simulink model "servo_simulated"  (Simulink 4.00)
settings: Solver=ode45  StartTime=0.0  StopTime=10  RelTol=1e-3
PreLoadFcn:
  | init_servo
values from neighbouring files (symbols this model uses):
  km = 2.96    [servo_model.m]    (also in init_servo.m; define_simulation_process.m)
libraries: cstblocks x3, simulink3 x3

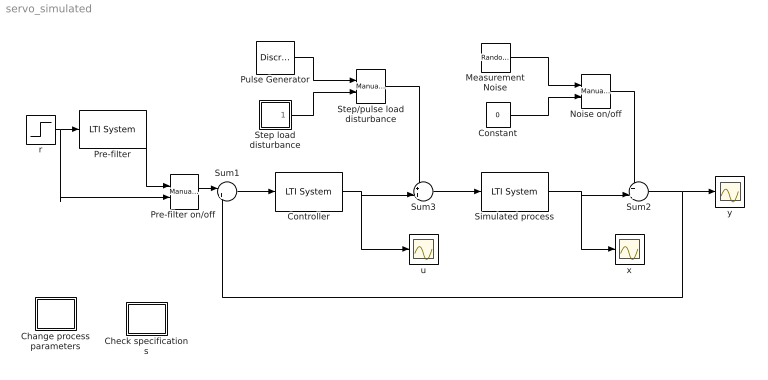
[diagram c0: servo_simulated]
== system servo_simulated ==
  Change process parameters : Subsystem
  Check specifications : Subsystem
  Constant : Constant  Value=0
  Controller : cstblocks/LTI System  sys=C  IC=[]
  Measurement Noise : RandomNumber  Mean=0  Variance=0.05*0.05  Seed=154542  SampleTime=0
  Noise on/off : simulink3/Nonlinear/Manual Switch  sw=1  action=0
  Pre-filter : cstblocks/LTI System  sys=F  IC=[]
  "Pre-filter on/off " : simulink3/Nonlinear/Manual Switch  sw=0  action=0
  Pulse Generator : DiscretePulseGenerator  PulseType=Time-based  Amplitude=-1  Period=100  PulseWidth=0.04  PhaseDelay=5  SampleTime=1
  Simulated process : cstblocks/LTI System  sys=P_sim  IC=[]
  Step load disturbance : Subsystem
  Step/pulse load disturbance : simulink3/Nonlinear/Manual Switch  sw=0  action=0
  Sum1 : Sum  Inputs=|+-  SaturateOnIntegerOverflow=on
  Sum2 : Sum  Inputs=++|  SaturateOnIntegerOverflow=on
  Sum3 : Sum  Inputs=++|  SaturateOnIntegerOverflow=on
  r : Step  Time=1  Before=0  After=5  SampleTime=0
  u : Scope
  x : Scope
  y : Scope
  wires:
  Sum1/1 -> Controller/1
  Controller/1 -> u/1, Sum3/2
  Sum3/1 -> Simulated process/1
  Simulated process/1 -> Sum2/2, x/1
  Constant/1 -> Noise on/off/2
  Measurement Noise/1 -> Noise on/off/1
  r/1 -> Pre-filter/1, "Pre-filter on/off "/2
  Step load disturbance/1(d) -> Step/pulse load disturbance/2
  Pulse Generator/1 -> Step/pulse load disturbance/1
  Step/pulse load disturbance/1 -> Sum3/1
  Noise on/off/1 -> Sum2/1
  Sum2/1 -> y/1, Sum1/2
  "Pre-filter on/off "/1 -> Sum1/1
  Pre-filter/1 -> "Pre-filter on/off "/1

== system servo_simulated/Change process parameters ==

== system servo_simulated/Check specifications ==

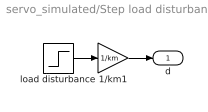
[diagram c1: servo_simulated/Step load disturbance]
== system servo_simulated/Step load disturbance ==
  1/km1 : Gain  Gain=1/km  Multiplication=Element-wise(K.*u)  SaturateOnIntegerOverflow=on
  load disturbance : Step  Time=5  Before=0  After=-0.15  SampleTime=0
  d : Outport  Port=1
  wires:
  load disturbance/1 -> 1/km1/1
  1/km1/1 -> d/1
